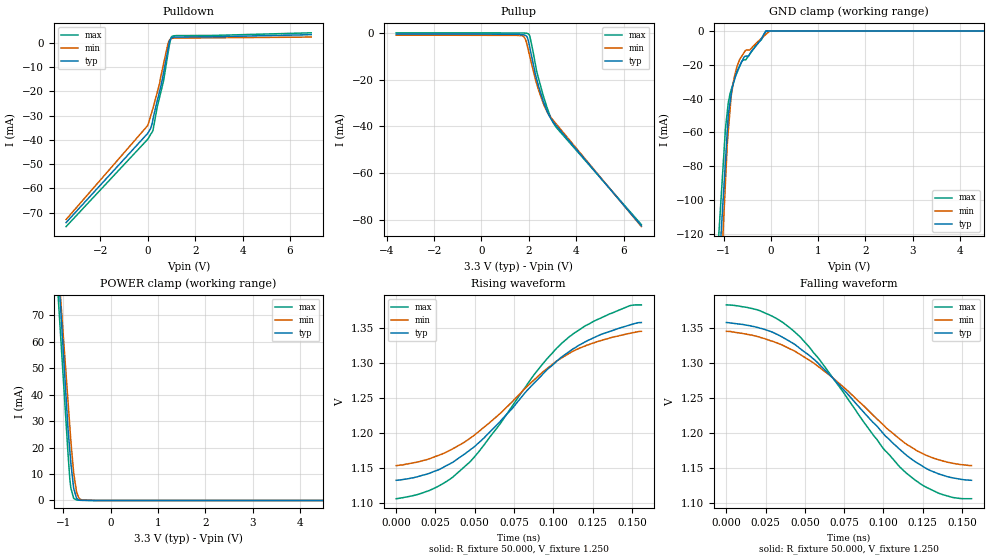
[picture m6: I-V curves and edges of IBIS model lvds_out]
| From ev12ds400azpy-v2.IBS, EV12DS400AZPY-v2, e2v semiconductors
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[Model]   lvds_out
Model_type Output
Vref=1.250E+00
Rref=5.000E+01
Cref=0.000E+00
Vmeas=1.250E+00
C_comp   6.720E-13   6.330E-13   7.190E-13
[Voltage Range]   3.300E+00   3.150E+00   3.450E+00
[POWER Clamp Reference]   3.300E+00   3.150E+00   3.450E+00
[GND Clamp Reference]   0.000E+00   0.000E+00   0.000E+00
[Pullup Reference]   3.300E+00   3.150E+00   3.450E+00
[Pulldown Reference]   0.000E+00   0.000E+00   0.000E+00
[Temperature Range]   25   110   -40
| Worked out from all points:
|   slope of the pulldown table from 0 to 0.495 V, typ, clamps not added: 28.8 ohm
|   slope of the pullup table from 0 to 0.495 V, typ, clamps not added: 41.2 kohm
|   GND clamp passes 1 mA (typ) near -0.13 V on its own axis
|   POWER clamp passes 1 mA (typ) near -0.72 V on its own axis
|   rising waveform, R_fixture 50.000, V_fixture 1.250: 20-80 % time 59.8ps typ, 58.5ps min, 57ps max; typ from 1.13 V to 1.36 V
|   falling waveform, R_fixture 50.000, V_fixture 1.250: 20-80 % time 58.2ps typ, 59.4ps min, 55.7ps max; typ from 1.36 V to 1.13 V
[GND Clamp]
-3.45V    -1.232A    -1.547A    -1.171A
-3.15V    -1.093A    -1.371A    -1.037A
-960mV    -77.45mA   -89.93mA   -58mA
-920mV    -58.91mA   -66.53mA   -47.68mA
-900mV    -49.64mA   -59.6mA    -42.52mA
-840mV    -37.84mA   -38.83mA   -35.02mA
-720mV    -24.06mA   -21.4mA    -25mA
-620mV    -18.46mA   -15.13mA   -18.23mA
-540mV    -14.97mA   -11.59mA   -17.06mA
-470mV    -14.85mA   -11.23mA   -14.66mA
-110mV    0A         -2.111mA   -518.8uA
6.9V      0A         0A         0A
[Pulldown]
-3.45V    -74.09mA   -72.82mA   -75.74mA
0V        -37.29mA   -34.05mA   -39.74mA
190mV     -33.09mA   -27.91mA   -36.74mA
220mV     -31.3mA    -26.94mA   -36.03mA
400mV     -23.78mA   -20.35mA   -26.38mA
500mV     -19.89mA   -16.7mA    -22.35mA
660mV     -12.58mA   -8.932mA   -15.9mA
840mV     -3.406mA   -864.9uA   -5.22mA
920mV     671.8uA    1.211mA    -473.8uA
980mV     1.864mA    1.653mA    2.04mA
1.04V     2.203mA    1.819mA    2.729mA
6.9V      3.333mA    2.347mA    4.1mA
[Pullup]
-3.6V     -517.6uA   -952.9uA   43.74uA
1.68V     -685.4uA   -1.139mA   -18.03uA
1.78V     -809.5uA   -1.476mA   -19.2uA
1.86V     -1.041mA   -2.798mA   -104.4uA
1.94V     -2.048mA   -5.84mA    -228uA
2V        -4.368mA   -8.373mA   -579uA
2.04V     -6.294mA   -10.06mA   -1.284mA
2.32V     -19.38mA   -21.43mA   -15.94mA
2.42V     -23.22mA   -24.76mA   -19.93mA
2.76V     -33.32mA   -33.66mA   -31.79mA
3.02V     -38.08mA   -37.39mA   -38.36mA
6.75V     -82.74mA   -83.04mA   -82.17mA
[POWER Clamp]
-3.6V     817mA      710.5mA    788.3mA
-3V       641.4mA    561mA      617mA
-1.02V    62.13mA    67.31mA    51.92mA
-900mV    27.02mA    37.39mA    17.68mA
-860mV    18.37mA    27.41mA    7.663mA
-840mV    14.05mA    22.43mA    4.76mA
-780mV    4.549mA    10.38mA    808.4uA
-720mV    846.6uA    3.275mA    173.1uA
-680mV    222.2uA    1.261mA    127.9uA
-640mV    50.39uA    438uA      112.2uA
-320mV    0A         10.14uA    0A
6.6V      0A         0A         0A
[Rising Waveform]
R_fixture = 50.000
V_fixture = 1.250
V_fixture_min = 1.250
V_fixture_max = 1.250
|  time   V(typ)   V(min)   V(max)
0s        1.133V     1.153V     1.106V
24ps      1.145V     1.166V     1.121V
36ps      1.158V     1.177V     1.137V
46.5ps    1.175V     1.192V     1.158V
66ps      1.216V     1.227V     1.212V
87.5ps    1.27V      1.275V     1.282V
110ps     1.316V     1.313V     1.337V
135.5ps   1.344V     1.335V     1.369V
148.5ps   1.354V     1.342V     1.381V
156ps     1.357V     1.345V     1.382V
[Falling Waveform]
R_fixture = 50.000
V_fixture = 1.250
V_fixture_min = 1.250
V_fixture_max = 1.250
|  time   V(typ)   V(min)   V(max)
0s        1.357V     1.345V     1.382V
21.5ps    1.349V     1.336V     1.374V
41.5ps    1.329V     1.319V     1.348V
52.5ps    1.311V     1.304V     1.323V
67.5ps    1.279V     1.279V     1.279V
99.5ps    1.2V       1.212V     1.179V
113ps     1.171V     1.187V     1.146V
124ps     1.154V     1.171V     1.127V
135ps     1.142V     1.162V     1.114V
156ps     1.133V     1.153V     1.106V
[Ramp]
| variable typ min max
dV/dt_r 145.848m/59.8950p 125.879m/58.5346p 161.561m/57.0117p
dV/dt_f 145.848m/58.1725p 125.879m/59.4632p 161.561m/55.7104p
R_load = 50.0000Ohms
